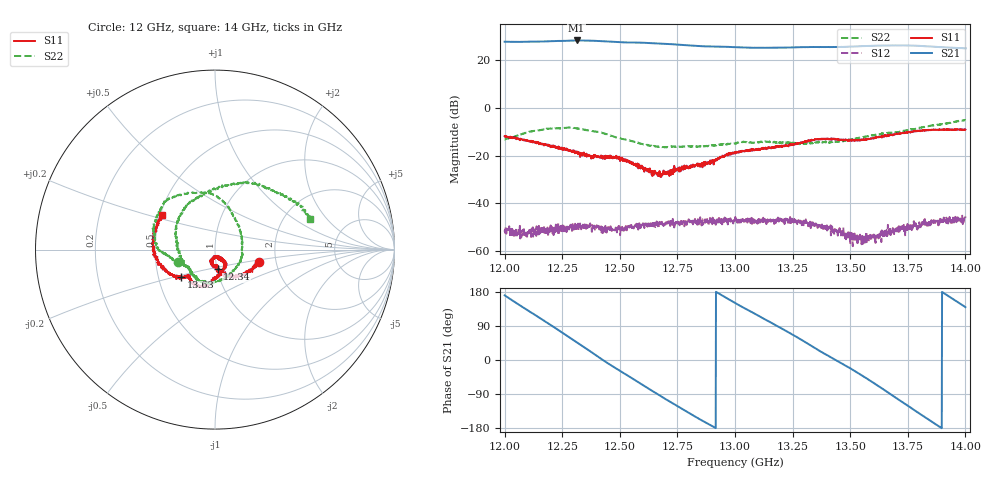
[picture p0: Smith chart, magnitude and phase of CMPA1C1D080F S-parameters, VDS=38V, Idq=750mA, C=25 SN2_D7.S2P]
!Keysight Technologies,E5071C,MY46632380,B.14.03
!Date: Thu Nov 05 05:02:56 2020
!Data & Calibration Information:
!Freq	S11:SOLT2(ON)	S21:SOLT2(ON)	S12:SOLT2(ON)	S22:SOLT2(ON)
!PortZ  Port1:50+j0  Port2:50+j0
!Above PortZ is port z conversion or system Z0 setting when saving the data.
!When reading, reference impedance value at option line is always used.
# Hz S dB R 50
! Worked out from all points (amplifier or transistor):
!   1601 points, 12 GHz to 14 GHz, reference 50 ohm
!   highest |S21| = 28.3 dB at 12.31 GHz (marker M1)
!   |S21| within 3 dB of that: start of sweep to 13.05 GHz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
!   unconditionally stable (mu >= 1): start of sweep to end of sweep
!   at 12.33 GHz: K = 5.94, MAG = 28.9 dB, |S12| = -50.9 dB
!   at 13 GHz: K = 6.39, MAG = 25.6 dB, |S12| = -47.9 dB
!   at 14 GHz: K = 3.28, MAG = 27.2 dB, |S12| = -45.5 dB
!   S11 on the Smith chart (normalised r, x): 12 GHz: 1.62, -0.24; 12.34 GHz: 1.00, -0.22; 13.63 GHz: 0.65, -0.21; 14 GHz: 0.51, +0.22
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1.2e10  -11.91 -15.8  27.75 170.6  -52.02 -147.8  -13.26 -161.6
1.208375e10  -13.69 -39.5  27.70 137.4  -50.93 -143.1  -10.72 -176.7
1.21725e10  -15.21 -61.6  27.87 103.1  -52.45 -130.9  -9.05 163.7
1.224e10  -17.13 -72.2  28.06 76.5  -49.75 -140.4  -8.67 147.0
1.23125e10  -18.92 -85.0  28.28 47.0  -50.74 -145.3  -8.64 127.9
1.233375e10  -18.99 -81.9  28.26 38.5  -49.69 -161.9  -8.99 120.7
1.233875e10  -19.11 -82.6  28.24 36.4  -49.89 -161.6  -8.97 118.8
1.24025e10  -20.62 -84.2  28.05 10.1  -50.44 -166.9  -10.04 94.9
1.246875e10  -20.94 -90.5  27.72 -16.7  -51.55 -173.4  -11.85 74.6
1.257875e10  -23.45 -102.6  27.38 -58.1  -48.55 -172.1  -14.68 44.1
1.26675e10  -28.37 -93.5  26.99 -91.3  -48.12 166.0  -16.14 11.2
1.2835e10  -24.06 -59.7  25.99 -152.1  -48.08 145.9  -16.17 -40.2
1.3e10  -19.18 -63.3  25.44 150.6  -47.92 117.9  -14.96 -90.8
1.317625e10  -16.70 -85.4  25.21 91.8  -48.37 78.1  -14.40 -124.8
1.333375e10  -13.70 -104.7  25.53 36.3  -48.57 35.6  -14.67 -150.2
1.34925e10  -13.45 -133.8  25.63 -19.3  -54.77 23.0  -13.27 174.3
1.36325e10  -12.24 -141.0  26.13 -72.9  -52.16 34.1  -11.00 128.2
1.36675e10  -11.51 -145.7  26.17 -87.1  -52.26 30.3  -10.49 117.3
1.374875e10  -10.12 -159.1  26.20 -120.3  -48.70 13.0  -9.46 88.6
1.383625e10  -9.29 -179.0  25.78 -155.5  -48.17 -1.1  -7.70 65.3
1.39125e10  -9.12 164.2  25.37 174.1  -46.98 -31.9  -6.67 44.2
1.4e10  -9.11 146.9  24.98 139.4  -45.52 -64.1  -5.12 18.1
